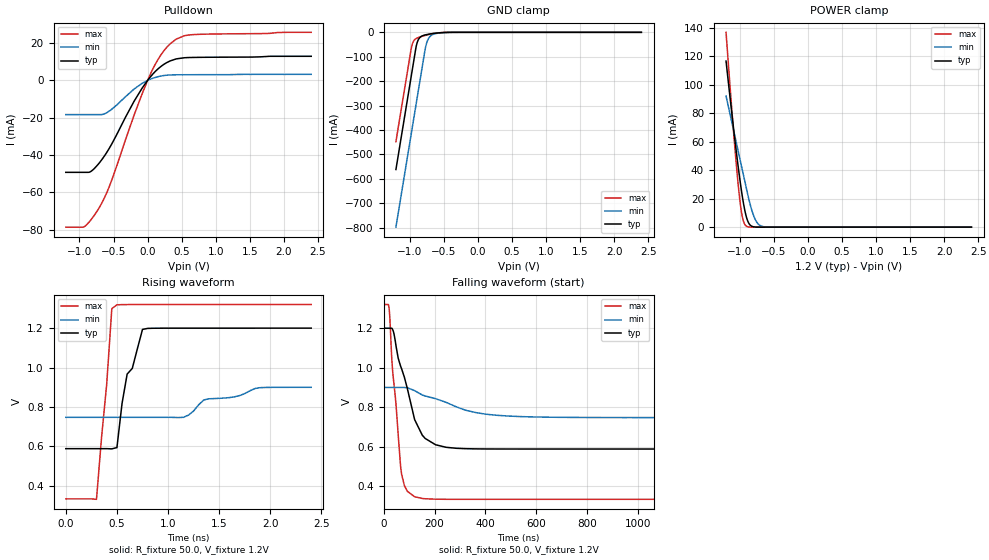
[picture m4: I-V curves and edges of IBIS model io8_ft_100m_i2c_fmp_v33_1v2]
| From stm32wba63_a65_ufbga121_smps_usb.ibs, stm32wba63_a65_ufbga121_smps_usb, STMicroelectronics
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[Model]   io8_ft_100m_i2c_fmp_v33_1v2
Model_type I/O_open_drain
Polarity   Non-Inverting
Enable   Active-Low
| CAP_THRESHOLD on pad IOFT is "UDTCAPC" :
| Rising=30.0% of vddiom   Falling=70.0% of vddiom
| C_comp min and max val. don't necessarily correlate with the min and max pvt
| but are the smallest and greatest pad capacitance found.
| var   typ   min   max
C_comp   2.88255pF  2.80651pF  2.98596pF
|C_comp_pulldown   2.88255pF  2.80651pF  2.98596pF
Vinl = 450.0mV
Vinh = 660.0mV
Vmeas = 600.0mV   | Reference voltage for timing measurements
Cref  = 50.0pF   | Timing specification test load capacitance value
Rref  = 1.0MOhm   | Timing specification test load resistance value
Vref  = 660.0mV   | Timing specification test load voltage
[Model Spec]
| TIME_THRESHOLD on pin ZII2CV11 is "CMOS" :
| Rising=50.0% of vdd   Falling=50.0% of vdd
Vinl 436.50000mV 331.50000mV 482.50000mV
Vinh 753.50000mV 549.50000mV 837.50000mV
| variable   typ   min   max
[Temperature Range] 25.0 140.0 -40.0
| variable   typ   min   max
[Voltage Range] 1.2V 900.0mV 1.32V
| variable   typ   min   max
[POWER Clamp Reference] 1.2V 900.0mV 1.32V
| variable   typ   min   max
[GND Clamp Reference] 0V 0V 0V
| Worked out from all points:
|   slope of the pulldown table from 0 to 0.18 V, typ, clamps not added: 25.7 ohm
|   GND clamp passes 1 mA (typ) near -0.51 V on its own axis
|   POWER clamp passes 1 mA (typ) near -0.83 V on its own axis
|   rising waveform, R_fixture 50.0, V_fixture 1.2V: 20-80 % time 165ps typ, 510ps min, 95.4ps max; typ from 0.588 V to 1.2 V
|   falling waveform, R_fixture 50.0, V_fixture 1.2V: 20-80 % time 78.7ns typ, 203ns min, 35.7ns max; typ from 1.2 V to 0.588 V
[POWER Clamp]
-1.2V     116.7mA    92.13mA    136.9mA
-1.09V    69.42mA    68.21mA    67.14mA
-1.02V    41.75mA    52.99mA    28.91mA
-990mV    30.98mA    46.47mA    16.09mA
-970mV    24.36mA    42.12mA    9.575mA
-940mV    15.59mA    35.6mA     3.485mA
-910mV    8.693mA    29.07mA    1.01mA
-860mV    2.259mA    18.59mA    104.6uA
-780mV    143.1uA    6.246mA    2.555uA
-720mV    16.22uA    1.846mA    157.1nA
-650mV    1.267uA    330.3uA    6.118nA
2.4V      0A         0A         0A
[GND Clamp]
-1.2V     -561.6mA   -797.4mA   -447.4mA
-980mV    -187.6mA   -423.4mA   -73.43mA
-960mV    -153.6mA   -389.4mA   -48.26mA
-900mV    -54.17mA   -287.4mA   -24.97mA
-870mV    -29.55mA   -236.4mA   -21.19mA
-830mV    -17.05mA   -168.4mA   -17.42mA
-760mV    -9.921mA   -54.55mA   -11.89mA
-730mV    -8.191mA   -29.78mA   -9.811mA
-690mV    -6.26mA    -14.49mA   -7.318mA
-600mV    -2.976mA   -4.315mA   -3.058mA
-380mV    -57.63uA   -251uA     -19.49uA
2.4V      872.8pA    204.8nA    349.4pA
| variable   typ   min   max
[Pullup Reference] 1.2V 900.0mV 1.32V
| variable   typ   min   max
[Pulldown Reference] 0V 0V 0V
[Pulldown]
-1.2V     -49.3mA    -18.35mA   -78.69mA
-930mV    -49.3mA    -18.35mA   -78.46mA
-830mV    -48.76mA   -18.35mA   -74.69mA
-700mV    -43.85mA   -18.35mA   -67.63mA
-540mV    -34.99mA   -15.84mA   -54.84mA
-200mV    -11.29mA   -4.684mA   -18.8mA
10mV      478.8uA    168.8uA    852.4uA
170mV     6.712mA    2.137mA    12.23mA
330mV     10.42mA    2.911mA    19.6mA
540mV     12.14mA    3.031mA    23.95mA
670mV     12.31mA    3.044mA    24.56mA
2.4V      12.92mA    3.23mA     25.77mA
[Ramp]
dV/dt_r 366.97124mV/3.19171ns 91.3824mV/10.19808ns 591.89479mV/1.63435ns
dV/dt_f 366.99016mV/76.76191ns 91.48132mV/203.22476ns 591.81479mV/35.37147ns
R_load = 50.0
| Removed startup time: 0s 0s 0s  .
| Removed end time: 2.4ns.
[Rising Waveform]
R_fixture   = 50.0
V_fixture   = 1.2V
V_fixture_min = 900.0mV
V_fixture_max = 1.32V
0s        588.3mV    747.5mV    333.6mV
300ps     588.4mV    747.5mV    331.3mV
400ps     588.4mV    747.5mV    915.6mV
450ps     587.4mV    747.5mV    1.299V
500ps     593.9mV    747.5mV    1.318V
600ps     967mV      747.5mV    1.32V
650ps     995.5mV    747.5mV    1.32V
750ps     1.194V     747.5mV    1.32V
1.85ns    1.2V       893.6mV    1.32V
2.4ns     1.2V       899.8mV    1.32V
| Removed startup time: 0s 0s 0s  .
| Removed end time: 1.99825us.
[Falling Waveform]
R_fixture   = 50.0
V_fixture   = 1.2V
V_fixture_min = 900.0mV
V_fixture_max = 1.32V
0s        1.2V       900mV      1.32V
21.75ns   1.2V       900mV      1.297V
35ns      1.194V     900mV      988.3mV
70.75ns   993.8mV    900mV      459.2mV
93ns      894.8mV    898.7mV    374.6mV
122.2ns   735.8mV    883.3mV    346.7mV
163.3ns   641.8mV    856.7mV    336.6mV
285.5ns   592.1mV    801.9mV    333.7mV
571ns     588.4mV    751.3mV    333.6mV
1.998us   588.3mV    747.5mV    333.6mV
